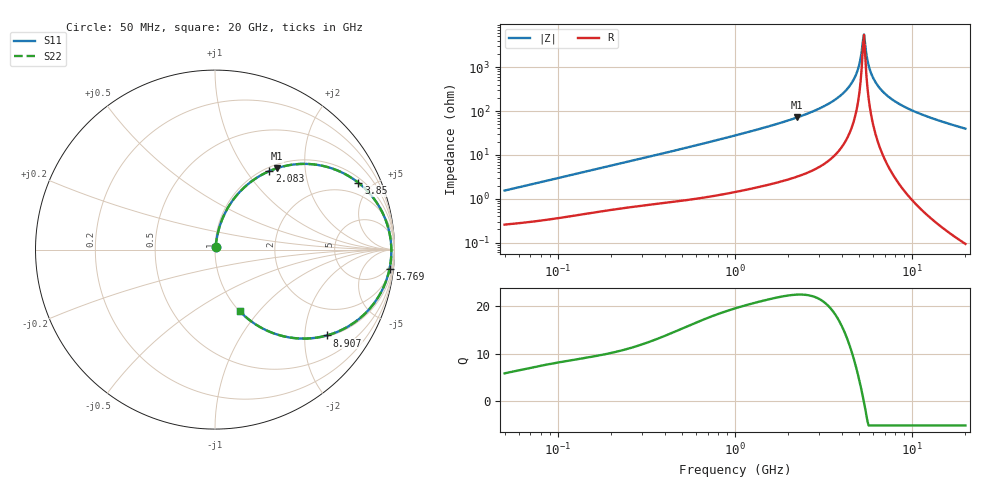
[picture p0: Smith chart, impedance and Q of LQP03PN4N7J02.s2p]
!Murata Part Number: LQP03PN4N7J02
!These Parameters are Measured in Series Mode Connection
!  o--[Z]--o
!Port1  Port2
!  o-------o
!Freq. Start=50[MHz] Stop=20[GHz], 401[Steps]
# Hz S RI R 50
!Freq.(Hz) S11(Real) S11(Imag) S21(Real) S21(Imag) S12(Real) S12(Imag) S22(Real) S22(Imag)
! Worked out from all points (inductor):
!   401 points, 50 MHz to 20 GHz, reference 50 ohm
!   read as one part in series: L = 4.77 nH near 51.52 MHz
!   highest Q = 22.3 at 2.245 GHz (marker M1), where L = 5.06 nH
!   self-resonance near 5.273 GHz
!   S11 on the Smith chart (normalised r, x): 50 MHz: 1.01, +0.03; 2.083 GHz: 1.06, +1.29; 3.85 GHz: 1.24, +4.16; 5.769 GHz: 3, -18; 8.907 GHz: 1.03, -2.59; 20 GHz: 1.00, -0.79
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5e7  0.00281 0.0151  0.9972 -0.0151  0.9972 -0.0151  0.00281 0.0151
1.364002e8  0.00591 0.0391  0.9941 -0.0391  0.9941 -0.0391  0.00591 0.0391
3.721004e8  0.0179 0.1  0.9821 -0.1  0.9821 -0.1  0.0179 0.1
1e9  0.0823 0.2503  0.9177 -0.2503  0.9177 -0.2503  0.0823 0.2503
1.498439e9  0.1676 0.3507  0.8324 -0.3507  0.8324 -0.3507  0.1676 0.3507
2.083303e9  0.302 0.4372  0.698 -0.4372  0.698 -0.4372  0.302 0.4372
2.245319e9  0.3449 0.4534  0.6551 -0.4534  0.6551 -0.4534  0.3449 0.4534
2.728004e9  0.4825 0.4775  0.5175 -0.4775  0.5175 -0.4775  0.4825 0.4775
3.850025e9  0.799 0.3724  0.201 -0.3724  0.201 -0.3724  0.799 0.3724
4.34015e9  0.8992 0.2642  0.1008 -0.2642  0.1008 -0.2642  0.8992 0.2642
4.748272e9  0.9533 0.1584  0.0467 -0.1584  0.0467 -0.1584  0.9533 0.1584
4.966507e9  0.9706 0.0995  0.0294 -0.0995  0.0294 -0.0995  0.9706 0.0995
5.194772e9  0.9805 0.0381  0.0195 -0.0381  0.0195 -0.0381  0.9805 0.0381
5.273168e9  0.982 0.0173  0.018 -0.0173  0.018 -0.0173  0.982 0.0173
5.433528e9  0.9824 -0.0245  0.0176 0.0245  0.0176 0.0245  0.9824 -0.0245
5.769027e9  0.9725 -0.1072  0.0275 0.1072  0.0275 0.1072  0.9725 -0.1072
6.034176e9  0.956 -0.167  0.044 0.167  0.044 0.167  0.956 -0.167
6.406762e9  0.9232 -0.2412  0.0768 0.2412  0.0768 0.2412  0.9232 -0.2412
7.442007e9  0.8011 -0.3874  0.1989 0.3874  0.1989 0.3874  0.8011 -0.3874
8.907419e9  0.6241 -0.4781  0.3759 0.4781  0.3759 0.4781  0.6241 -0.4781
1.314879e10  0.3116 -0.4607  0.6884 0.4607  0.6884 0.4607  0.3116 -0.4607
2e10  0.1366 -0.3423  0.8634 0.3423  0.8634 0.3423  0.1366 -0.3423
